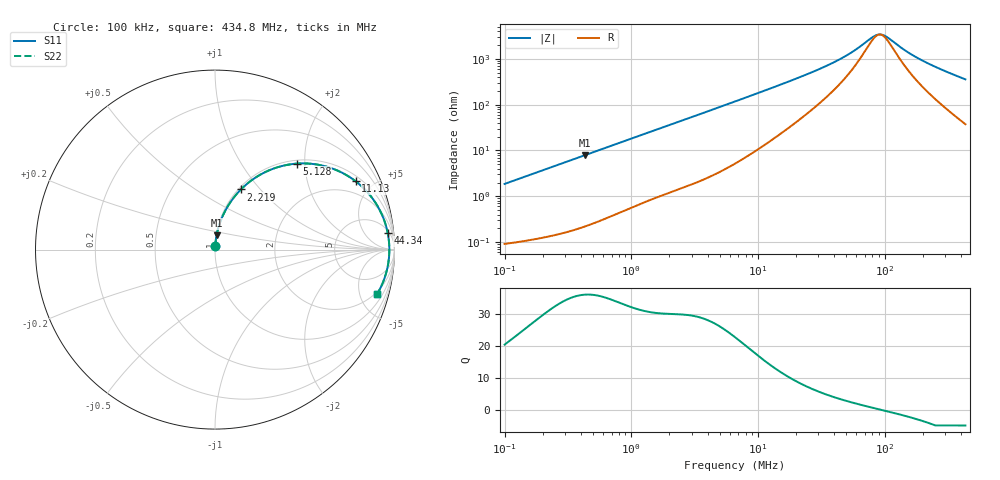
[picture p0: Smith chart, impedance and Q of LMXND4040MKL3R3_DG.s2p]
! LMXND4040MKL3R3_DG  S-PARAMETER MODEL  ( General Type )
! Model Generated by TAIYO YUDEN Corporation (http://www.ty-top.com)
! Version 1.0
! TAIYO YUDEN Control No. 191023NI43SB-FBB
! Copyright(c) 2019 TAIYO YUDEN CO.,LTD. All Rights Reserved.
! Product Description (link to TY-COMPAS)
! https://ds.yuden.co.jp/TYCOMPAS/or/detail?pn=LMXND4040MKL3R3MDG&u=M
! Products Name : Inductors
! Characteristics :
!  Inductance : 3.3 uH , SRF(min) : 60 MHz , DC Resistance(max) : 0.084 Ohm
!  Rated Current : Saturation :1400 mA , Temp Rise : 1700 mA
!  Case Size : 4.0 x 4.0 / 0.157 x 0.157 [mm/inch] , Thickness : 1.2 / 0.047 [mm/inch]
!  (Conditions: Temperature = 25 degC , DC Bias Current/Voltage = 0A / 0V)
! External Node Assignments :
!  1  o---GGG---o  2
! GND o---------o GND
! Frequency Range : 0.1MHz  -  434.768421MHz  [ 402 STEP ]
# MHz S RI R 50
! Freq[MHz].  S11 Real  S11 Imag  S21 Real  S21 Imag  S12 Real  S12 Imag  S22 Real  S22 Imag
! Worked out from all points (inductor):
!   401 points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, 100 kHz to 434.8 MHz, reference 50 ohm
!   read as one part in series: L = 2.96 uH near 104.3 kHz
!   highest Q = 36.1 at 433.2 kHz (marker M1), where L = 2.92 uH
!   self-resonance near 91.78 MHz
!   S11 on the Smith chart (normalised r, x): 100 kHz: 1.00, +0.04; 2.219 MHz: 1.03, +0.79; 5.128 MHz: 1.07, +1.82; 11.13 MHz: 1.26, +3.98; 44.34 MHz: 7, +19; 434.8 MHz: 1.75, -7.08
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0.1  0.00126 0.0186  0.9987 -0.0186  0.9987 -0.0186  0.00126 0.0186
0.406826  0.0076 0.0741  0.9924 -0.0741  0.9924 -0.0741  0.0076 0.0741
0.433207  0.00845 0.0787  0.9915 -0.0787  0.9915 -0.0787  0.00845 0.0787
0.864672  0.0286 0.1522  0.9714 -0.1522  0.9714 -0.1522  0.0286 0.1522
1.65507  0.0888 0.2683  0.9112 -0.2683  0.9112 -0.2683  0.0888 0.2683
2.218991  0.1442 0.3349  0.8558 -0.3349  0.8558 -0.3349  0.1442 0.3349
3.303488  0.2638 0.4239  0.7362 -0.4239  0.7362 -0.4239  0.2638 0.4239
5.128392  0.455 0.479  0.545 -0.479  0.545 -0.479  0.455 0.479
6.733248  0.585 0.4709  0.415 -0.4709  0.415 -0.4709  0.585 0.4709
11.13064  0.7841 0.3805  0.2159 -0.3805  0.2159 -0.3805  0.7841 0.3805
16.57057  0.8797 0.2821  0.1203 -0.2821  0.1203 -0.2821  0.8797 0.2821
26.82484  0.938 0.1758  0.062 -0.1758  0.062 -0.1758  0.938 0.1758
44.34378  0.9626 0.0915  0.0374 -0.0915  0.0374 -0.0915  0.9626 0.0915
57.01386  0.9679 0.0573  0.0321 -0.0573  0.0321 -0.0573  0.9679 0.0573
84.8785  0.9713 0.00911  0.0287 -0.00911  0.0287 -0.00911  0.9713 0.00911
90.38256  0.9714 0.00178  0.0286 -0.00178  0.0286 -0.00178  0.9714 0.00178
96.24353  0.9714 -0.00553  0.0286 0.00553  0.0286 0.00553  0.9714 -0.00553
109.1303  0.971 -0.0203  0.029 0.0203  0.029 0.0203  0.971 -0.0203
146.3135  0.9682 -0.0561  0.0318 0.0561  0.0318 0.0561  0.9682 -0.0561
192.1002  0.9624 -0.0932  0.0376 0.0932  0.0376 0.0932  0.9624 -0.0932
285.9862  0.9449 -0.1583  0.0551 0.1583  0.0551 0.1583  0.9449 -0.1583
434.7684  0.9048 -0.2454  0.0952 0.2454  0.0952 0.2454  0.9048 -0.2454
